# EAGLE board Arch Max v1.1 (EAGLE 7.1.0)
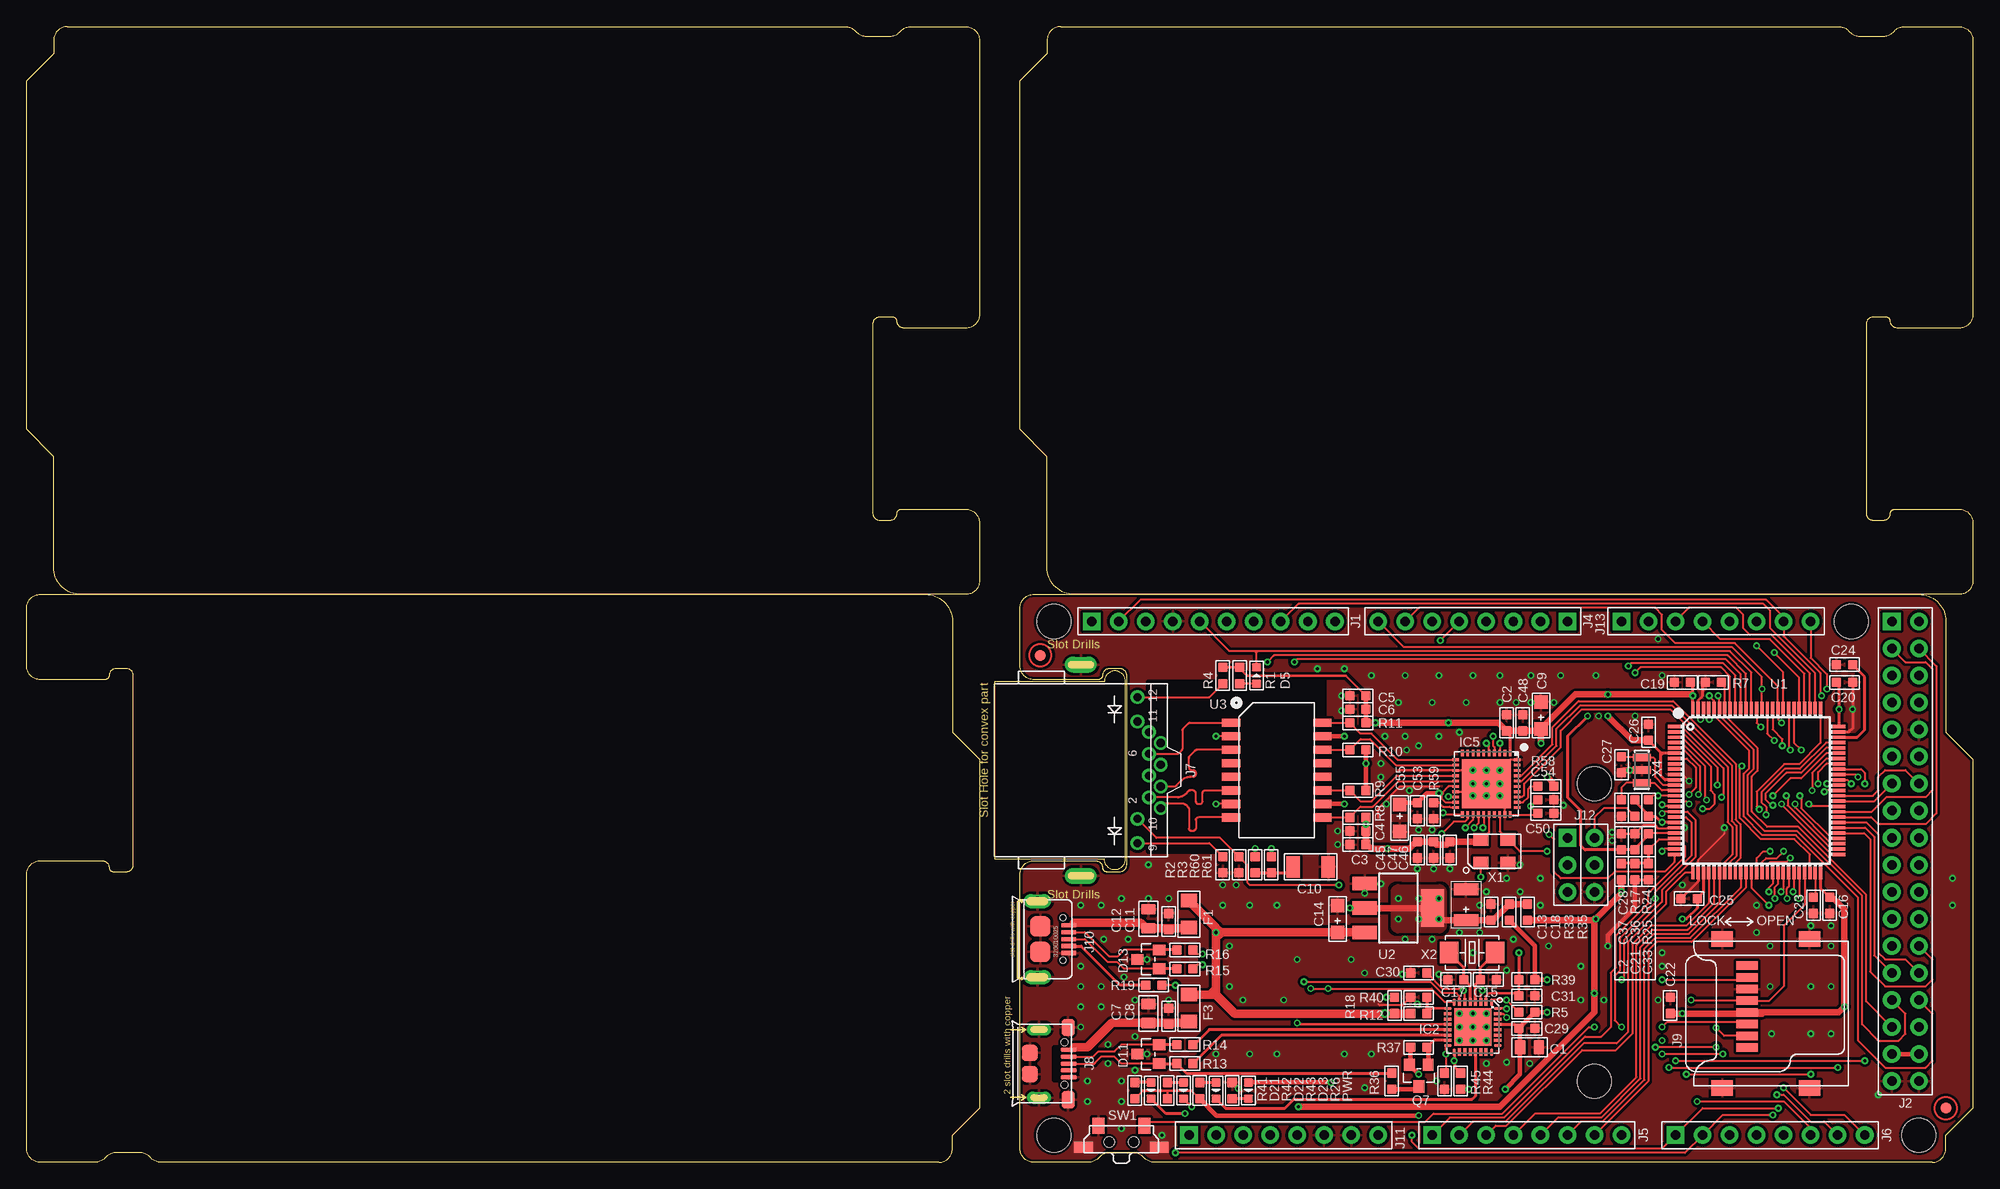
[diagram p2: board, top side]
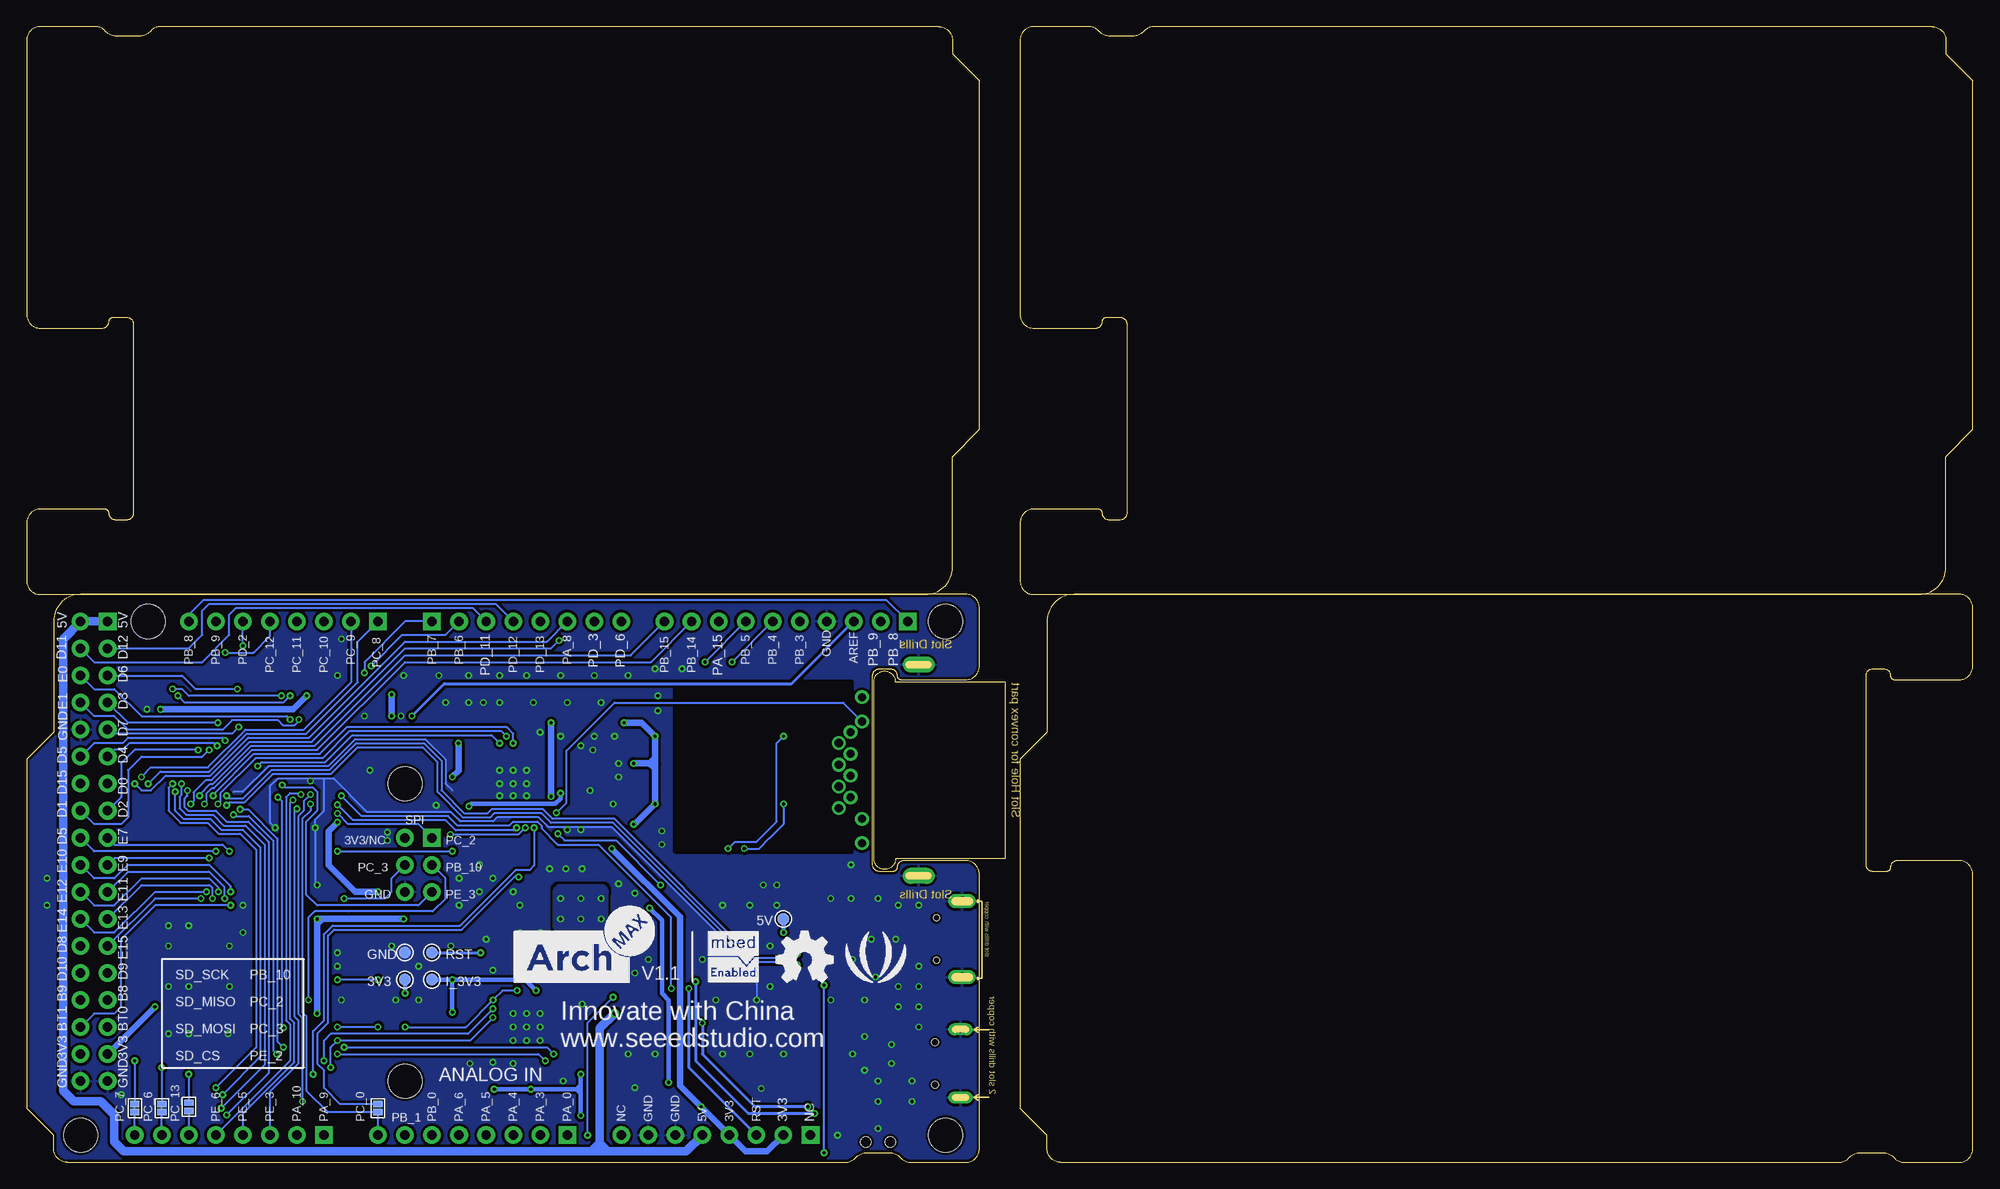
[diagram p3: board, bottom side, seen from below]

Size 182.88 x 106.68 mm. Coordinates in mm from the lower left corner, seen from the top.
Outline: 136 segments
Copper layers (1*16): Top 0.035mm / dielectric 1.5mm / Bottom 0.035mm
Design rules "SeeedStudio_2layer_DRU_no_angle_20140221 *": minimum track width 6mil, minimum drill 12mil, track to track 6mil, track to pad 6mil, pad to pad 6mil, via to via 6mil, smd to smd 0mil, copper to edge 10mil, drill to drill 10mil, minimum pad ring 10mil, minimum via ring 6mil, stop-mask expansion 2mil, vias tented up to drill 100mil, thermal gap 10mil
Net classes: 0 default: width 0.102 mm, drill 0.203 mm, clearance 0.102 mm
Holes 3.2 mm at 171.45,50.8 177.8,2.54 147.32,35.56 96.52,50.8 96.52,2.54 147.32,7.62
Holes 1.91 mm at 2.54,-6.35 180.34,-6.35 2.54,113.03 180.34,113.03
tRestrict: area 105.4,29.2 to 121.9,45.1
bRestrict: area 105.4,29.2 to 121.9,45.1

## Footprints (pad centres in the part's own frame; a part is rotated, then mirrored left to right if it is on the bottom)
TP_4545 = smd 1.143 x 1.143: T 0,0
C0805 = smd 1.016 x 1.397: 1 -0.889,0; 2 0.889,0
C0603 = smd 0.889 x 0.889: 1 -0.762,0; 2 0.762,0
AVX-A = smd 1.27 x 1.27: + -1.27,0; - 1.27,0
C1206 = smd 1.27 x 2.032: 1 -1.651,0; 2 1.651,0
AVX-B = smd 1.143 x 2.286: + -1.46,0; - 1.46,0
LED-0603 = smd 0.762 x 0.889: + -0.762,0; - 0.762,0
SOT23 = smd 1.016 x 1.143: 1 -0.889,-1.016; 2 0.889,-1.016; 3 0,1.016
F1206 = smd 1.27 x 1.524: 1 -1.27,0; 2 1.27,0
MBED-ICS_HVQFN33 = smd 0.7 x 0.28: 1 -2.35,1.75; 2 -2.35,1.25; 3 -2.35,0.75; 4 -2.35,0.25; 5 -2.35,-0.25; 6 -2.35,-0.75; 7 -2.35,-1.25; 8 -2.35,-1.75; 17 2.35,-1.75; 18 2.35,-1.25; 19 2.35,-0.75; 20 2.35,-0.25; 21 2.35,0.25; 22 2.35,0.75; 23 2.35,1.25; 24 2.35,1.75 | smd 0.28 x 0.7: 9 -1.75,-2.35; 10 -1.25,-2.35; 11 -0.75,-2.35; 12 -0.25,-2.35; 13 0.25,-2.35; 14 0.75,-2.35; 15 1.25,-2.35; 16 1.75,-2.35; 25 1.75,2.35; 26 1.25,2.35; 27 0.75,2.35; 28 0.25,2.35; 29 -0.25,2.35; 30 -0.75,2.35; 31 -1.25,2.35; 32 -1.75,2.35 | smd 3.5 x 3.5: EXP 0,0
LLP-40 = smd 0.25 x 0.6: 1 2.25,2.9; 2 1.75,2.9; 3 1.25,2.9; 4 0.75,2.9; 5 0.25,2.9; 6 -0.25,2.9; 7 -0.75,2.9; 8 -1.25,2.9; 9 -1.75,2.9; 10 -2.25,2.9; 21 -2.25,-2.9; 22 -1.75,-2.9; 23 -1.25,-2.9; 24 -0.75,-2.9; 25 -0.25,-2.9; 26 0.25,-2.9; 27 0.75,-2.9; 28 1.25,-2.9; 29 1.75,-2.9; 30 2.25,-2.9 | smd 0.6 x 0.25: 11 -2.9,2.25; 12 -2.9,1.75; 13 -2.9,1.25; 14 -2.9,0.75; 15 -2.9,0.25; 16 -2.9,-0.25; 17 -2.9,-0.75; 18 -2.9,-1.25; 19 -2.9,-1.75; 20 -2.9,-2.25; 31 2.9,-2.25; 32 2.9,-1.75; 33 2.9,-1.25; 34 2.9,-0.75; 35 2.9,-0.25; 36 2.9,0.25; 37 2.9,0.75; 38 2.9,1.25; 39 2.9,1.75; 40 2.9,2.25 | smd 4.6 x 4.6: DAP 0,0
10P-2.54-65/35MIL = drill 0.889 pad 1.651 square: 1 0,11.43 | drill 0.889 pad 1.651: 2 0,8.89; 3 0,6.35; 4 0,3.81; 5 0,1.27; 6 0,-1.27; 7 0,-3.81; 8 0,-6.35; 9 0,-8.89; 10 0,-11.43
2.54-2X18P = drill 0.889 pad 1.651 square: 1 -1.27,21.59 | drill 0.889 pad 1.651: 2 -1.27,19.05; 3 -1.27,16.51; 4 -1.27,13.97; 5 -1.27,11.43; 6 -1.27,8.89; 7 -1.27,6.35; 8 -1.27,3.81; 9 -1.27,1.27; 10 -1.27,-1.27; 11 -1.27,-3.81; 12 -1.27,-6.35; 13 -1.27,-8.89; 14 -1.27,-11.43; 15 -1.27,-13.97; 16 -1.27,-16.51; 17 -1.27,-19.05; 18 -1.27,-21.59; 19 1.27,-21.59; 20 1.27,-19.05; 21 1.27,-16.51; 22 1.27,-13.97; 23 1.27,-11.43; 24 1.27,-8.89; 25 1.27,-6.35; 26 1.27,-3.81; 27 1.27,-1.27; 28 1.27,1.27; 29 1.27,3.81; 30 1.27,6.35; 31 1.27,8.89; 32 1.27,11.43; 33 1.27,13.97; 34 1.27,16.51; 35 1.27,19.05; 36 1.27,21.59
CK_1X8 = drill 0.889 pad 1.651 square: 1 0,8.89 | drill 0.889 pad 1.651: 2 0,6.35; 3 0,3.81; 4 0,1.27; 5 0,-1.27; 6 0,-3.81; 7 0,-6.35; 8 0,-8.89
RJ45-MJ88-BX11-RVSL2 = drill 0.762 pad 1.27: 1 3.57,7.5; 2 2.55,6.4; 3 1.53,7.5; 4 0.51,6.4; 5 -0.51,7.5; 6 -1.53,6.4; 7 -2.55,7.5; 8 -3.57,6.4; 9 6.86,5.32; 10 4.57,5.32; 11 -4.57,5.32; 12 -6.86,5.32 | drill 0.6 pad 1.5 long: 13 -9.92,0; 14 9.92,0
MICRO-USB = smd 0.381 x 1.524: 1 -1.3,-0.25; 2 -0.65,-0.25; 3 0,-0.25; 4 0.65,-0.25; 5 1.3,-0.25 | smd 1.6 x 1.2: S1 -3.4,-0.3; S6 3.4,-0.3 | drill 0.635 pad 1.143 long: S2 -3.2,-3.048; S5 3.2,-3.048 | smd 1.5 x 1.5: S3 -1,-3.9; S4 1,-3.9 | hole 0.635: -2,-0.65; 2,-0.65
8P-SMD = smd 0.8 x 2.008: 1 -3.198,0.254; 2 -2.098,0.254; 3 -0.998,0.254; 4 0.102,0.254; 5 1.202,0.254; 6 2.302,0.254; 7 3.402,0.254; 8 4.502,0.254 | smd 1.45 x 2: 9 -7.002,2.6; 10 7.002,2.6; 11 -7.002,-5.598; 12 7.002,-5.598
MICRO-USB-5P-AB = smd 0.4 x 1.35: 1 -1.3,2.675; 2 -0.65,2.675; 3 0,2.675; 4 0.65,2.675; 5 1.3,2.675 | smd 1.9 x 1.9: P1 -1.2,0; P2 1.2,0 | drill 0.8 pad 1.2 long: P3 -3.575,-0.265; P4 3.575,-0.265 | hole 0.55: -2,2.15; 2,2.15
2X3P-2.54-65/35MIL = drill 0.889 pad 1.651 square: 1 -1.27,2.54 | drill 0.889 pad 1.651: 2 -1.27,0; 3 -1.27,-2.54; 4 1.27,-2.54; 5 1.27,0; 6 1.27,2.54
L0603 = smd 0.889 x 0.889: 1 -0.762,0; 2 0.762,0
2P-SMD-1.78X1.27 = smd 0.889 x 0.61: 1 0,0.381; 2 0,-0.381
ROUND-MARK-1.0 = smd 1.016 x 1.016: P$1 0,0
R0603 = smd 0.889 x 0.889: 1 -0.762,0; 2 0.762,0
4P-SMD-7X3.5X3.5H = smd 1.143 x 1.524: 1 -2.159,1.524; 2 2.159,1.524 | smd 1.778 x 1.016: S1 -3.556,-0.508; S2 3.556,-0.508 | hole 0.95: -1.15,0; 1.15,0
LQFP100 = smd 1.2 x 0.32: 1 -7.75,6; 2 -7.75,5.5; 3 -7.75,5; 4 -7.75,4.5; 5 -7.75,4; 6 -7.75,3.5; 7 -7.75,3; 8 -7.75,2.5; 9 -7.75,2; 10 -7.75,1.5; 11 -7.75,1; 12 -7.75,0.5; 13 -7.75,0; 14 -7.75,-0.5; 15 -7.75,-1; 16 -7.75,-1.5; 17 -7.75,-2; 18 -7.75,-2.5; 19 -7.75,-3; 20 -7.75,-3.5; 21 -7.75,-4; 22 -7.75,-4.5; 23 -7.75,-5; 24 -7.75,-5.5; 25 -7.75,-6; 51 7.75,-6; 52 7.75,-5.5; 53 7.75,-5; 54 7.75,-4.5; 55 7.75,-4; 56 7.75,-3.5; 57 7.75,-3; 58 7.75,-2.5; 59 7.75,-2; 60 7.75,-1.5; 61 7.75,-1; 62 7.75,-0.5; 63 7.75,0; 64 7.75,0.5; 65 7.75,1; 66 7.75,1.5; 67 7.75,2; 68 7.75,2.5; 69 7.75,3; 70 7.75,3.5; 71 7.75,4; 72 7.75,4.5; 73 7.75,5; 74 7.75,5.5; 75 7.75,6 | smd 0.32 x 1.2: 26 -6,-7.75; 27 -5.5,-7.75; 28 -5,-7.75; 29 -4.5,-7.75; 30 -4,-7.75; 31 -3.5,-7.75; 32 -3,-7.75; 33 -2.5,-7.75; 34 -2,-7.75; 35 -1.5,-7.75; 36 -1,-7.75; 37 -0.5,-7.75; 38 0,-7.75; 39 0.5,-7.75; 40 1,-7.75; 41 1.5,-7.75; 42 2,-7.75; 43 2.5,-7.75; 44 3,-7.75; 45 3.5,-7.75; 46 4,-7.75; 47 4.5,-7.75; 48 5,-7.75; 49 5.5,-7.75; 50 6,-7.75; 76 6,7.75; 77 5.5,7.75; 78 5,7.75; 79 4.5,7.75; 80 4,7.75; 81 3.5,7.75; 82 3,7.75; 83 2.5,7.75; 84 2,7.75; 85 1.5,7.75; 86 1,7.75; 87 0.5,7.75; 88 0,7.75; 89 -0.5,7.75; 90 -1,7.75; 91 -1.5,7.75; 92 -2,7.75; 93 -2.5,7.75; 94 -3,7.75; 95 -3.5,7.75; 96 -4,7.75; 97 -4.5,7.75; 98 -5,7.75; 99 -5.5,7.75; 100 -6,7.75
SOT-223 = smd 1.27 x 2.286: 1 -2.286,-3.175; 2 0,-3.175; 3 2.286,-3.175 | smd 3.556 x 2.159: TER 0,3.175
SOIC16-9.53 = smd 0.762 x 1.714: 1 -4.445,-4.286; 2 -3.175,-4.286; 3 -1.905,-4.286; 4 -0.635,-4.286; 5 0.635,-4.286; 6 1.905,-4.286; 7 3.175,-4.286; 8 4.445,-4.286; 9 4.445,4.286; 10 3.175,4.286; 11 1.905,4.286; 12 0.635,4.286; 13 -0.635,4.286; 14 -1.905,4.286; 15 -3.175,4.286; 16 -4.445,4.286
4P-SMD-5X3.2 = smd 1.4 x 1.2: 1 -1.27,-1.1; 2 1.27,-1.1; 3 1.27,1.1; 4 -1.27,1.1
2P-SMD-5X3.2 = smd 1.778 x 2.032: 1 -2.159,0; 2 2.159,0
3P-SMD-3.6X1.3 = smd 0.7 x 1.7: 1 -1.2,0; 2 0,0; 3 1.2,0

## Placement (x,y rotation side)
3V3  NC  [TP_4545]  147.32,17.14 270 bottom
5V  NC  [TP_4545]  111.76,22.86 270 bottom
C1  10uF  [C0805]  141.22,10.79 180 top
C2  100nF  [C0603]  139.06,41.27 270 top
C3  100nF  [C0603]  125.09,29.84 180 top
C4  100nF  [C0603]  125.09,31.11 180 top
C5  100nF  [C0603]  125.09,43.81 180 top
C6  100nF  [C0603]  125.09,42.55 180 top
C7  10uF  [C0805]  105.41,13.97 90 top
C8  100nF  [C0603]  107.31,13.72 90 top
C9  16V 10uF  [AVX-A]  142.3,41.97 90 top
C10  1000v_1nF  [C1206]  120.65,27.75 180 top
C11  100nF  [C0603]  107.31,22.61 90 top
C12  10uF  [C0805]  105.41,22.86 90 top
C13  10V 47uF  [AVX-B]  135.25,24.19 90 top
C14  10uF/16v  [AVX-A]  123.19,22.86 90 top
C15  18pF  [C0603]  137.35,17.14 180 top
C16  100nF  [C0603]  169.42,24.13 90 top
C17  18pF  [C0603]  134.3,17.14 0 top
C18  100nF  [C0603]  137.6,23.5 270 top
C19  100nF  [C0603]  155.57,45.09 0 top
C20  100nF  [C0603]  170.81,45.09 180 top
C21  100nF  [C0603]  151.13,27.3 90 top
C22  100nF  [C0603]  154.43,14.73 90 top
C23  2.2uF  [C0603]  167.89,24.13 90 top
C24  2.2uF  [C0603]  170.81,46.74 0 top
C25  100nF  [C0603]  156.21,24.77 0 top
C26  100nF  [C0603]  152.4,40.39 270 top
C27  DNP  [C0603]  149.86,37.34 90 top
C28  DNP  [C0603]  149.86,33.27 90 top
C29  100nF  [C0603]  140.97,12.57 180 top
C30  100nF  [C0603]  130.81,17.78 0 top
C31  100nF  [C0603]  140.97,15.62 180 top
C33  1uF  [C0603]  152.4,27.3 90 top
C36  1uF  [C0603]  151.13,30.1 270 top
C37  100nF  [C0603]  149.86,30.1 270 top
C45  100nF  [C0603]  130.68,29.34 90 top
C46  100nF  [C0603]  133.73,29.34 90 top
C47  100nF  [C0603]  132.21,29.34 270 top
C48  100nF  [C0603]  140.59,41.27 90 top
C50  100nF  [C0603]  142.75,32.77 0 top
C53  100nF  [C0603]  130.68,33.02 90 top
C54  100nF  [C0603]  142.75,34.04 180 top
C55  16V 10uF  [AVX-A]  129.03,32.32 270 top
D5  GREEN  [LED-0603]  115.57,45.72 90 top
D11  CESD3V3AP  [SOT23]  105.41,10.16 90 top
D13  CESD3V3AP  [SOT23]  105.41,19.05 90 top
D21  RED  [LED-0603]  105.66,6.73 270 top
D22  BULE  [LED-0603]  108.71,6.73 270 top
D23  YELLOW  [LED-0603]  111.76,6.73 270 top
F1  PPTC_750mA  [F1206]  109.22,23.3 90 top
F3  PPTC_750mA  [F1206]  109.22,14.48 90 top
GND  NC  [TP_4545]  147.32,19.68 270 bottom
I_3V3  NC  [TP_4545]  144.78,17.14 270 bottom
IC2  LPC11U35FHI33/501  [MBED-ICS_HVQFN33]  135.89,12.7 270 top
IC5  DP83848J  [LLP-40]  137.16,35.56 0 top
J1  320030059  [10P-2.54-65/35MIL]  111.51,50.8 90 top
J2  DNP/2.54 Female 2*18p  [2.54-2X18P]  176.53,29.21 0 top
J4  2.54 female 8p  [CK_1X8]  135.89,50.8 270 top
J5  2.54 female 8p  [CK_1X8]  140.97,2.54 90 top
J6  2.54 female 8p  [CK_1X8]  163.83,2.54 90 top
J7  RJ45-MJ88-BX11-RVSL2  [RJ45-MJ88-BX11-RVSL2]  99.06,36.83 270 top
J8  340005001  [MICRO-USB]  98.17,9.27 270 top
J9  320090002  [8P-SMD]  161.93,13.97 90 top
J10  320010025  [MICRO-USB-5P-AB]  95.25,20.95 270 top
J11  2.54 female 8p  [CK_1X8]  118.11,2.54 90 top
J12  320020027  [2X3P-2.54-65/35MIL]  146.05,27.94 0 top
J13  2.54 female 8p  [CK_1X8]  158.75,50.8 90 top
L2  120R-500mA  [L0603]  149.86,27.3 270 top
P1  NC  [2P-SMD-1.78X1.27]  167.64,5.21 180 bottom
P2  NC  [ROUND-MARK-1.0]  not placed on the board
P3  NC  [ROUND-MARK-1.0]  not placed on the board
P4  NC  [ROUND-MARK-1.0]  not placed on the board
P5  NC  [2P-SMD-1.78X1.27]  149.86,5.08 180 bottom
P6  NC  [ROUND-MARK-1.0]  180.34,5.08 0 top
P7  NC  [ROUND-MARK-1.0]  95.25,47.62 0 top
P8  NC  [ROUND-MARK-1.0]  not placed on the board
P9  NC  [2P-SMD-1.78X1.27]  170.18,5.08 0 bottom
P10  NC  [2P-SMD-1.78X1.27]  172.72,5.08 180 bottom
PWR  Green  [LED-0603]  114.81,6.73 270 top
Q7  CJ2305  [SOT23]  130.81,8.13 180 top
R1  470R  [R0603]  113.98,45.72 90 top
R2  470R  [R0603]  112.39,27.94 90 top
R3  2.2K  [R0603]  113.92,27.94 90 top
R4  470R  [R0603]  112.39,45.72 270 top
R5  DNP  [R0603]  140.97,14.1 0 top
R7  10K  [R0603]  158.5,45.09 0 top
R8  49.9R_1%  [R0603]  125.09,32.38 180 top
R9  49.9R_1%  [R0603]  125.09,34.92 0 top
R10  49.9R_1%  [R0603]  125.09,38.73 180 top
R11  49.9R_1%  [R0603]  125.09,41.27 0 top
R12  10k  [R0603]  130.81,13.97 180 top
R13  33R  [R0603]  108.84,9.27 180 top
R14  33R  [R0603]  108.84,11.05 180 top
R15  33R  [R0603]  108.84,18.16 180 top
R16  33R  [R0603]  108.84,19.94 180 top
R17  DNP  [R0603]  151.13,33.27 90 top
R18  10k  [R0603]  128.52,14.73 270 top
R19  0R  [R0603]  105.92,16.64 180 top
R24  10K  [R0603]  152.4,33.27 270 top
R25  0R  [R0603]  152.4,30.1 270 top
R26  470R  [R0603]  113.28,6.73 270 top
R33  0R  [R0603]  139.32,23.5 270 top
R35  0R  [R0603]  141.03,23.5 90 top
R36  1.5k  [R0603]  128.27,7.62 90 top
R37  DNP  [R0603]  130.81,10.79 180 top
R39  10k  [R0603]  140.97,17.14 0 top
R40  100k  [R0603]  130.81,15.49 0 top
R41  470R  [R0603]  104.14,6.73 270 top
R42  470R  [R0603]  107.19,6.73 270 top
R43  470R  [R0603]  110.24,6.73 270 top
R44  DNP  [R0603]  134.75,7.62 270 top
R45  DNP  [R0603]  133.22,7.62 90 top
R58  2.2K  [R0603]  142.75,35.31 180 top
R59  4.87K_1%  [R0603]  132.21,33.02 270 top
R60  75R  [R0603]  115.44,27.94 90 top
R61  75R  [R0603]  116.97,27.94 90 top
RST  NC  [TP_4545]  144.78,19.68 0 bottom
SW1  BUTTON-4P-REINFORCE'TS-1188E'  [4P-SMD-7X3.5X3.5H]  102.87,1.91 0 top
U1  STM32F407VET6  [LQFP100]  162.56,34.92 0 top
U2  CJT1117-3.3  [SOT-223]  128.91,23.88 270 top
U3  HX1198NL  [SOIC16-9.53]  117.47,36.83 270 top
U$1  [SEEEDSTUDIO-PCB-FRAME]  not placed on the board
U$2  [SEEEDSTUDIO-PCB-FRAME]  not placed on the board
U$3  [SEEEDSTUDIO-PCB-FRAME]  not placed on the board
U$4  [SEEEDSTUDIO-PCB-FRAME]  not placed on the board
U$5  [SEEEDSTUDIO-PCB-FRAME]  not placed on the board
X1  50MHz/052012001  [4P-SMD-5X3.2]  137.92,29.21 0 top
X2  12MHz/050016001  [2P-SMD-5X3.2]  135.83,19.68 0 top
X4  8MHz  [3P-SMD-3.6X1.3]  151.76,36.83 270 top

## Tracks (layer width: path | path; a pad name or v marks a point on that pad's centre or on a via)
50MHZ  (via drill 0.3 pad 0.64)
  Top 0.203: IC5.28 138.41,31.09 X1.3 140.29,29.21 v142.88,29.21 | U1.24 153.88,29.43 v153.67,29.21
  Bottom 0.203: v153.67,29.21 v142.88,29.21
+3.3V  (via drill 0.3 pad 0.64)
  Top 0.203: IC5.18 133.65,34.31 v133.6,34.35 | IC5.26 137.41,32.7 137.41,30.99 136.74,30.31 X1.4 | 170.31,45.08 C20.2 | 151.13,33.91 R17.2
  Top 0.254: R4.1 R1.2 113.98,46.42 114.68,45.72 123.95,45.72 C5.1
  Top 0.305: U1.28 157.56,25.35 C25.2 156.97,23.88 155.96,22.86 v155.57,22.86 | U1.100 v156.56,43.81 156.56,44.86 C19.2 | U1.75 v170.31,42.54 170.31,45.08 | R24.2 152.4,32.38 | R17.2 151.13,34.16 | U1.50 168.56,25.75 C16.2 | IC5.1 139.41,40.26 | 139.41,40.26 139.41,40.8 | 151.13,33.91 152.4,32.64 R24.2 | C2.2 139.16,40.51 139.41,40.26 | U1.6 153.74,38.42 | 153.74,38.42 153.6,38.42 | 153.6,38.42 153.54,38.48 | 153.54,38.48 C26.2 | U1.11 153.94,35.92 153.54,36.32 153.54,38.23 | 153.54,38.23 153.54,38.37 | 153.54,38.37 153.6,38.42 | 153.54,38.37 153.54,38.48 | U1.19 153.66,31.93 | R24.2 153.03,32.51 153.62,31.93 153.66,31.93 | 153.74,38.42 153.54,38.23 | 153.66,31.93 v153.67,31.94
  Top 0.406: C5.1 C6.1 R11.2 | R10.1 v125.86,37.47 R9.2 | U3.10 v123.82,33.66 | v123.82,40.01 U3.15 | 130.43,29.84 C45.2 130.56,30.1 | J2.20 J2.17 | C25.2 156.97,24.64 | 136.55,30.2 X1.4
  Top 0.61: R11.2 v126.75,41.27 v133.6,41.27 138.3,41.27 C2.2 C48.1 142.11,40.51 C9.+ | C16.2 169.67,24.89 170.81,23.75 v170.81,14.61 170.28,14.07 163.19,14.07 | J9.4 163.19,14.07 | 163.19,14.07 163.09,13.97 v155.57,13.97 C22.1 | C9.+ v142.3,39.37 | C9.+ 145.54,43.94 v148.59,43.94 156.43,43.94 v156.56,43.81 | v147.45,22.86 147.32,22.86 147.32,22.73 | 147.32,22.48 v147.32,15.88 147.32,14.1 138.43,5.21 v119.51,5.21 | 147.32,22.48 147.32,22.73 | 147.32,22.48 147.07,22.73 | R8.1 v125.86,31.75 C4.1 125.86,29.97 | 125.86,29.97 C3.1 | 125.86,29.97 126.36,29.46 v127.89,29.46 129.92,29.46 130.56,30.1 | C45.2 C47.1 132.46,29.84 133.48,29.84 C46.2 136.44,30.1 136.55,30.2 | L2.2 v149.86,25.4 149.86,25.27 v147.45,22.86 | R35.1 147.32,22.73 | 147.32,22.73 v147.45,22.86 | R58.1 143.51,35.56 v142.88,36.2 | C26.2 150.88,39.62 v148.59,41.91
  Bottom 0.406: 3V3.T v147.32,15.88
  Bottom 0.61: 123.82,37.47 v123.82,33.66 125.73,31.75 v125.86,31.75 | 123.82,37.47 v123.82,40.01 125.09,41.27 v126.75,41.27 | v125.86,37.47 124.46,37.47 | 124.46,37.47 123.82,37.47 | J2.17 v170.81,14.61 | 124.46,37.47 arc-45 124.24,37.55 123.95,37.85 | 124.46,37.47 arc45 124.24,37.38 123.95,37.08 | v170.31,42.54 157.83,42.54 v156.56,43.81 | v127.89,29.46 121.48,23.05 121.48,7.18 v119.51,5.21 J11.4 115.32,1.02 113.28,1.02 J11.2 | v133.6,34.35 v133.6,41.27 | v142.3,39.37 142.3,36.77 v142.88,36.2 | v148.59,41.91 v148.59,43.94 | v153.67,31.94 154.5,31.11 154.5,27.88 152.02,25.4 v149.86,25.4 | v147.45,22.86 155.07,22.86 | 155.07,22.86 155.45,22.86 | v155.57,13.97 155.57,22.35 | 155.57,22.35 v155.57,22.86 | 155.07,22.86 155.57,22.35
AREF  (via drill 0.3 pad 0.64)
  Top 0.203: U1.21 152.72,30.93 152.65,30.86 R25.1
  Top 0.305: R25.1 152.4,30.73 151.13,29.46 C36.2 C37.2 146.43,29.34 146.05,29.72 146.05,33.02 144.78,34.29 144.78,40.01 v146.69,41.91
  Bottom 0.305: v146.69,41.91 143.64,44.96 111,44.96 J1.3
BOOT0
  Top 0.203: J2.16 172.85,15.11 172.85,25.15 166.5,31.5 163.54,31.5 162.11,32.93 162.11,36.25 162.62,36.77 162.62,38.92 159.56,41.99 U1.94 159.56,45.04 159.51,45.09 R7.2
BOOT1  (via drill 0.3 pad 0.64)
  Top 0.203: U1.37 162.06,25.77 v163.7,24.13
  Bottom 0.203: v163.7,24.13 170.81,24.13 173.99,20.95 173.99,14.61 174.62,13.97 176.53,13.97 J2.21
DB_RX  (via drill 0.3 pad 0.64)
  Top 0.203: v154.94,9.53 v172.72,9.53
  Top 0.254: IC2.32 139.03,14.45 v139.06,14.41
  Bottom 0.203: v139.06,14.41 141.41,12.06 154.31,12.06 154.94,11.43 v154.94,9.53 | v172.72,9.53 P10.2
DB_TX  (via drill 0.3 pad 0.64)
  Top 0.203: IC2.31 138.7,13.95 v139.06,13.59 | v154.31,8.89 v170.18,8.89
  Bottom 0.203: v139.06,13.59 141.22,11.43 v153.67,11.43 154.31,10.79 v154.31,8.89 | v170.18,8.89 P9.1
ETH_CRS_DV
  Top 0.203: U1.32 159.56,28.18 160.27,28.89 160.27,31.5 159.83,31.94 159.83,37.15 154.43,42.55 146.15,42.55 144.14,40.54 144.14,38.99 140.72,35.56 140.72,34.54 140.48,34.31 IC5.33
ETH_MDC  (via drill 0.3 pad 0.64)
  Top 0.203: U1.16 153.84,33.42 v153.67,33.59 | IC5.25 136.91,31.5 v136.84,31.43
  Bottom 0.203: v136.84,31.43 137.1,31.18 142.56,31.18 143.51,32.13 152.21,32.13 v153.67,33.59
ETH_MDIO  (via drill 0.3 pad 0.64)
  Top 0.203: IC5.24 136.41,31.83 v136.02,31.43 | U1.25 154.81,28.19 153.92,27.3 149.22,27.3 148.59,26.67 144.14,26.67 143.51,27.3 143.51,30.35 v143.06,30.8
  Bottom 0.203: v136.02,31.43 136.65,30.8 v143.06,30.8
ETH_RX_D0
  Top 0.203: IC5.36 140.46,35.81 143.76,39.12 143.76,40.7 145.99,42.93 154.58,42.93 160.21,37.3 160.21,32.07 160.66,31.62 160.66,28.77 160.06,28.17 U1.33
ETH_RX_D1
  Top 0.203: U1.34 160.56,28.1 161.04,28.57 161.04,31.75 160.59,32.19 160.59,37.43 154.71,43.31 145.81,43.31 143.38,40.88 143.38,39.24 140.45,36.31 IC5.37
ETH_TX_D0  (via drill 0.3 pad 0.64)
  Top 0.203: U1.51 169.58,28.93 164.91,33.59 v164.91,33.66 | v137.79,40.01 137.79,39.12 137.92,38.99 137.92,38.47 IC5.4
  Bottom 0.203: v164.91,33.66 164.68,33.88 164.68,34.65 161.36,37.97 155.07,37.97 152.53,40.51 138.3,40.51 v137.79,40.01
ETH_TX_D1  (via drill 0.3 pad 0.64)
  Top 0.203: U1.52 169.58,29.43 165.48,33.53 165.48,34.29 v165.35,34.42 | IC5.5 137.41,39.12 v137.16,39.37
  Bottom 0.203: v137.16,39.37 137.16,40.26 137.79,40.89 152.78,40.89 155.32,38.35 161.54,38.35 165.35,34.54 v165.35,34.42
ETH_TX_EN  (via drill 0.3 pad 0.64)
  Top 0.203: U1.48 167.56,28.91 166.12,30.35 162.96,30.35 160.97,32.35 160.97,37.02 v161.16,37.21 | v138.43,39.37 138.43,38.48 IC5.3
  Bottom 0.203: v161.16,37.21 160.78,37.59 154.81,37.59 152.27,40.13 139.19,40.13 v138.43,39.37
FSMC_D0
  Top 0.203: U1.61 173.62,33.92 J2.7
FSMC_D1
  Top 0.203: U1.62 173.49,34.42 173.99,34.92 173.99,36.2 174.62,36.83 176.53,36.83 J2.30
FSMC_D2  (via drill 0.3 pad 0.64)
  Top 0.203: U1.81 166.06,39.43 v166.75,38.73
  Bottom 0.203: J2.8 173.99,34.29 173.99,37.47 172.72,38.73 v166.75,38.73
FSMC_D3  (via drill 0.3 pad 0.64)
  Top 0.203: U1.82 165.56,38.91 v165.74,38.73
  Bottom 0.203: J2.29 176.53,31.75 173.99,31.75 173.35,32.38 173.35,36.83 172.08,38.1 166.37,38.1 v165.74,38.73
FSMC_D4  (via drill 0.3 pad 0.64)
  Top 0.203: U1.38 162.56,28.57 163.19,29.21 v163.83,29.21
  Bottom 0.203: J2.9 174.62,29.84 164.46,29.84 v163.83,29.21
FSMC_D5  (via drill 0.3 pad 0.64)
  Top 0.203: U1.39 163.06,28.19 163.45,28.57 164.46,28.57 v165.1,29.21
  Bottom 0.203: v165.1,29.21 176.53,29.21 J2.28
FSMC_D6  (via drill 0.3 pad 0.64)
  Top 0.203: U1.40 163.56,27.92 163.83,28.19 165.35,28.19 v165.74,28.57
  Bottom 0.203: v165.74,28.57 174.62,28.57 J2.10
FSMC_D7  (via drill 0.3 pad 0.64)
  Top 0.203: v163.7,25.4 163.7,25.78 164.06,26.14 U1.41
  Bottom 0.203: J2.27 176.53,26.67 174.62,26.67 173.35,27.94 165.74,27.94 163.7,25.91 v163.7,25.4
FSMC_D8  (via drill 0.3 pad 0.64)
  Top 0.203: v164.27,24.77 164.27,25.84 164.56,26.13 U1.42
  Bottom 0.203: v164.27,24.77 164.27,25.84 165.74,27.3 173.35,27.3 J2.11
FSMC_D9  (via drill 0.3 pad 0.64)
  Top 0.203: U1.43 165.06,25.61 v164.85,25.4
  Bottom 0.203: J2.26 176.53,24.13 174.62,24.13 172.08,26.67 165.74,26.67 164.85,25.78 v164.85,25.4
FSMC_D10  (via drill 0.3 pad 0.64)
  Top 0.203: v165.42,24.77 165.42,25.72 165.56,25.86 U1.44
  Bottom 0.203: v165.42,24.77 165.42,25.72 165.74,26.04 172.08,26.04 J2.12
FSMC_D11  (via drill 0.3 pad 0.64)
  Top 0.203: U1.45 166.06,25.47 v165.99,25.4
  Bottom 0.203: J2.25 176.53,21.59 174.62,21.59 170.81,25.4 v165.99,25.4
FSMC_D12  (via drill 0.3 pad 0.64)
  Top 0.203: v166.5,24.77 166.62,24.89 166.62,27.11 U1.46
  Bottom 0.203: v166.5,24.77 170.81,24.77 J2.13
FSMC_D13
  Top 0.203: U1.55 172.66,30.93 173.23,30.35 173.23,17.91 174.62,16.51 178.44,16.51 179.07,17.14 179.07,19.05 J2.24
FSMC_D14
  Top 0.203: U1.56 172.75,31.43 173.61,30.57 173.61,19.43 J2.14
FSMC_D15
  Top 0.203: U1.57 172.86,31.93 173.99,30.79 173.99,19.68 174.62,19.05 176.53,19.05 J2.23
FSMC_NBL0  (via drill 0.3 pad 0.64)
  Top 0.203: U1.97 158.06,41.65 v158.12,41.59
  Bottom 0.203: J2.34 176.53,44.45 174.62,44.45 172.08,41.91 158.43,41.91 v158.12,41.59
FSMC_NBL1  (via drill 0.3 pad 0.64)
  Top 0.203: U1.98 157.56,41.86 v157.29,41.59
  Bottom 0.203: J2.33 176.53,41.91 174.62,41.91 173.35,40.64 164.46,40.64 163.58,41.53 159.26,41.53 158.75,41.02 157.73,41.02 157.29,41.47 v157.29,41.59
FSMC_NE1/NCE2  (via drill 0.3 pad 0.64)
  Top 0.203: U1.88 | U1.88 162.56,42.74 162.5,42.8 | U1.88 162.56,41.27 v162.94,40.89
  Bottom 0.203: J2.5 174.88,40.26 163.58,40.26 v162.94,40.89
FSMC_NOE  (via drill 0.3 pad 0.64)
  Top 0.203: U1.85 164.06,40.66 164.97,39.75 v164.97,39.12
  Bottom 0.203: J2.6 174.62,38.73 173.86,38.73 173.23,39.37 165.23,39.37 v164.97,39.12
FSMC_NWE  (via drill 0.3 pad 0.64)
  Top 0.203: 163.58,42.67 163.57,42.67 U1.86 163.56,40.27 v164.21,39.62
  Bottom 0.203: J2.31 176.53,39.37 173.86,39.37 173.35,39.88 164.46,39.88 v164.21,39.62
GND  (via drill 0.3 pad 0.64)
  Top 0.203: 128.91,36.83 128.93,36.81 IC5.13 135.87,36.81 135.87,37.45 | 132.72,35.31 129.03,35.31 127,33.27 127,32.38 | C37.1 C36.1 151.95,31.69 152.97,31.69 153.29,31.37 154.75,31.37 U1.20 155.76,31.43 v155.76,31.43 | IC5.17 135.37,34.81 | IC5.29 138.91,33.81 | IC5.40 139.41,37.81 v138.43,36.83 | 135.37,35.04 v135.89,35.56 | U1.10 155.6,36.42 v156.21,35.81 | v159.51,31.43 159.51,30.86 157.06,28.41 U1.27 | R40.1 129.29,14.73 127.13,14.73 127,14.86 | v130.68,14.86 130.3,15.24
  Top 0.254: R26.1 v113.85,6.92 114.05,6.73 | C21.1 151.13,26.67
  Top 0.305: U1.99 157.06,43.4 157.48,43.81 157.48,44.83 R7.1 | C20.1 171.58,40.77 171.24,40.42 U1.74 | U1.27 157.06,26.38 C25.1 | C21.1 C33.1
  Top 0.406: 135.37,34.81 135.37,35.04 | v148.59,20.32 148.59,21.34 151.13,23.88 C21.1
  Top 0.61: X4.2 150.11,36.83 C27.1
  Bottom 0.203: 163.45,34.8 162.56,34.8 160.15,37.21 154.56,37.21 152.02,39.75 145.41,39.75 143.51,37.85 143.51,35.57 142.86,34.92 | 154.94,36.07 159.26,36.07 160.02,35.31 160.02,31.94 v159.51,31.43 | 154.94,36.07 154.05,36.07 150.88,32.89 143,32.89 142.12,32.01 139.06,32.01 138.68,32.38 134.75,32.38 133.86,31.5 127.89,31.5 114.3,17.91 v114.3,15.24 | v155.57,26.04 155.76,26.23 v155.76,31.43 155.76,32.19 154.94,33.02 154.94,36.07
  other vias: 105.28,19.05 99.69,7.62 105.28,10.16 99.69,5.71 132.46,7.62 134.62,13.97 135.89,13.97 137.16,13.97 137.16,12.7 137.16,11.43 135.89,11.43 134.62,11.43 134.62,12.7 135.89,12.7 141.22,9.27 139.06,18.03 173.99,6.35 163.96,12.06 167.64,12.06 163.83,16.51 169.55,22.23 167.64,22.23 153.29,15.24 135.89,36.83 137.16,36.83 138.43,35.56 137.16,35.56 127.25,37.47 127.63,40.01 129.67,38.73 123.57,42.42 123.57,43.81 132.72,40.01 129.54,40.01 142.24,26.67 111.76,10.16 114.94,10.16 117.47,10.16 139.06,9.4 137.16,9.27 153.67,45.72 171.58,42.55 153.29,49.15 127.25,36.2 129.92,34.92 107.31,15.24 105.41,24.77 107.31,24.77 112.39,26.04 113.66,26.04 138.43,43.18 143.51,43.18 141.35,43.18 139.95,43.18 130.68,27.56 132.21,27.56 133.73,27.56 130.81,39.12 127.76,33.66 139.06,26.67 125.73,25.27 125.73,17.78 136.53,24.13 148.97,30.23 132.72,17.65 126.36,10.16 113.03,16.51 180.97,26.67 180.97,24.13 129.54,45.72 128.91,43.18 135.25,43.18 125.73,6.99 153.67,19.68 153.67,18.41 124.46,19.05 119.38,19.05 118.11,15.24 113.03,20.32 123.82,10.16 129.29,17.65 99.06,18.41 103.12,17.4 100.97,24.13 99.06,24.13 105.41,27.94 112.39,24.13 127.25,26.16 123.19,31.11 123.19,29.84 130.81,31.24 132.08,31.24 126.36,45.72 132.72,45.72 135.89,45.72 138.43,45.72 141.35,45.72 144.14,45.72 147.45,45.72 121.28,46.35 123.82,46.35 142.24,24.13 140.33,25.4 146.05,18.41 143,20.32 139.7,20.95 129.54,20.95 134.62,40.39 135.89,34.42 137.16,34.42 138.43,34.42 162.56,21.59 163.83,20.32 169.55,20.32 167.64,16.51 169.55,16.51 169.55,12.06 150.62,36.83 148.97,30.99 144.4,33.53 151.13,41.91 147.7,41.91 117.47,24.13 114.94,24.13 134.62,21.59 136.53,21.59 135.89,19.68 132.08,20.95 146.05,15.24 148.21,15.24 137.16,25.4 140.33,27.94 102.87,3.17 106.68,2.54 104.14,8.64 102.87,5.71 100.97,16.51 99.06,16.51 99.06,12.7 99.06,14.61 100.97,14.61 101.6,11.05 104.14,15.24 101.22,20.95 103.5,20.95 102.87,24.77 101.6,9.27 104.14,11.81 102.87,7.62 162.56,24.13 132.08,43.18
  pour Bottom (isolate 0.254, rank 6): 93.34,53.34 182.88,53.34 182.88,0 93.34,0
  pour Top (isolate 0.254, rank 6): 93.34,53.34 182.88,53.34 182.88,0 93.34,0
GREEN  (via drill 0.3 pad 0.64)
  Top 0.254: IC2.12 119.51,12.95 v119.38,13.08
  Top 0.305: v109.47,5.21 D22.-
  Bottom 0.305: v119.38,13.08 119.38,10.16 114.43,5.21 v109.47,5.21
GREEN1  (via drill 0.3 pad 0.64)
  Top 0.203: IC2.7 134.64,15.6 134.37,15.88 132.97,15.88 131.89,16.95 v120.02,16.95
  Top 0.305: v108.84,4.57 107.06,4.57 D21.-
  Bottom 0.305: v120.02,16.95 120.02,9.53 115.06,4.57 v108.84,4.57
I2C1_SCL  (via drill 0.3 pad 0.64)
  Top 0.203: v158.94,43.81 159.06,43.7 U1.95 159.06,41.98 162.24,38.8 162.24,36.89 161.75,36.4 161.75,32.7 163.33,31.11 166.37,31.11 172.47,25.02 172.47,12.95 173.99,11.43 175.89,11.43 176.53,12.06 176.53,13.97 J2.15 | J13.8 167.64,47.37 169.16,45.85 v169.16,44.45
  Bottom 0.203: v158.94,43.81 167.64,43.81 168.27,44.45 v169.16,44.45 | J13.8 167.64,51.44 166.24,52.83 102.11,52.83 J1.1
I2C1_SDA  (via drill 0.3 pad 0.64)
  Top 0.203: v158.12,43.81 158.56,43.37 U1.96 158.56,41.97 161.86,38.67 161.86,37.02 161.35,36.51 161.35,32.49 163.11,30.73 166.24,30.73 172.08,24.89 172.08,11.45 174.64,8.89 178.44,8.89 179.07,9.53 179.07,13.97 J2.22 | v168.66,43.81 168.53,43.94 168.53,45.97 165.1,49.4 J13.7 165.1,51.18 163.45,52.83 104.65,52.83 J1.2
  Bottom 0.203: v158.12,43.81 158.75,43.18 168.02,43.18 v168.66,43.81
ID
  Top 0.305: R19.2 102.74,16.64 99.08,20.3 J10.4
LED_LINK  (via drill 0.3 pad 0.64)
  Top 0.203: v123.32,26.04 114.94,26.04 114.68,26.29 114.68,27.94 R3.2 112.14,30.48 106.16,30.48 J7.10 | IC5.22 135.41,32.29 135.13,32 134.11,32 v132.97,30.86
  Bottom 0.203: v123.32,26.04 127.51,30.23 132.33,30.23 v132.97,30.86
LED_SPEED  (via drill 0.3 pad 0.64)
  Top 0.203: IC5.21 133.26,32.66 v133.1,32.83
  Bottom 0.203: v133.1,32.83 132.14,33.78 132.14,38.67 127.63,43.18 106.16,43.18 J7.11
N$1
  Top 0.305: J10.1 98.39,22.25 98.42,22.23 98.42,22.48
  Top 0.813: 107.44,21.97 C12.1 105.16,21.97 104.65,22.48 98.42,22.48 | 107.44,21.97 109.16,21.97 F1.1 | C11.1 107.44,21.97
N$2
  Top 0.203: R17.1 150.37,33.27 148.21,33.27 147.32,32.38 J12.6
N$3  (via drill 0.3 pad 0.64)
  Top 0.203: R5.1 v139.06,15.24 137.83,15.24 IC2.1 | v147.32,12.7 146.81,12.7 138.68,4.57 132.21,4.57 131.44,3.81 105.41,3.81 SW1.2 | IC2.3 136.64,15.99 v136.78,16.13
  Bottom 0.203: v147.32,12.7 141.6,12.7 v139.06,15.24 138.17,16.13 v136.78,16.13
N$4  (via drill 0.3 pad 0.64)
  Top 0.203: IC5.23 135.91,32.15 v135.19,31.43 | v155.96,8.26 v167.64,8.26
  Bottom 0.203: v135.19,31.43 135.19,27.88 135.64,27.43 136.94,27.43 142.15,22.23 154.14,22.23 154.94,21.42 154.94,13.34 155.96,12.32 v155.96,8.26 | v167.64,8.26 P1.2
N$5
  Top 0.254: IC2.9 131.6,14.45 131.57,14.48
  Top 0.305: R40.2 131.57,14.48 R12.1
N$6
  Top 0.203: J7.9 111.13,29.97 R2.2
N$7
  Top 0.203: J7.12 111.13,43.69 R4.2
N$8
  Top 0.203: D5.+ R1.1
N$9  (via drill 0.3 pad 0.64)
  Top 0.203: v136.65,26.8 X1.1
  Bottom 0.203: v136.65,26.8 137.03,26.8 141.99,21.84 153.99,21.84 154.56,21.28 154.56,13.08 155.57,12.06 155.57,9.27 154.94,8.64 154.94,6.99 153.42,5.46 P5.2
N$10
  Top 0.203: J8.1 98.2,10.57 98.42,10.79
  Top 0.305: 98.45,10.82 98.42,10.79
  Top 0.813: 107.44,13.08 C7.1 101.98,13.08 99.69,10.79 98.42,10.79 | F3.1 109.09,13.08 107.44,13.08 | 107.44,13.08 C8.1
N$12
  Top 0.305: IC2.14 112.28,11.95 R13.1
N$13
  Top 0.305: IC2.13 111.13,12.45 109.73,11.05 R14.1
N$15
  Top 0.203: D13.1 103.12,18.16 102.49,18.8 101.6,18.8 99.44,20.95 J10.3
  Top 0.305: R15.2 D13.1
N$18
  Top 0.305: PWR.- R26.2
N$22
  Top 0.203: D13.2 103.12,19.94 102.49,19.3 101.73,19.3 99.43,21.61 J10.2
  Top 0.305: R16.2 D13.2
N$23  (via drill 0.3 pad 0.64)
  Top 0.406: PWR.+ v122.55,7.49 | U2.2 125.22,23.88 125.09,23.75 | C18.2 137.67,22.73
  Top 0.61: C13.+ 135.89,22.73 136.02,22.61 135.38,22.61 C13.+ | C13.+ C18.2 137.79,22.73 R33.1 R35.2 | C13.+ 132.33,22.73 132.08,22.99 U2.TER U2.2 v124.33,23.88
  Bottom 0.406: v122.55,7.49 122.55,15.24 123.19,15.88 123.19,22.73 v124.33,23.88
  other vias: 128.91,24.77 132.72,24.77 132.72,22.86 130.81,22.86 130.81,24.77 128.91,22.86
  pour Top (isolate 0.254, no thermals): 132.72,21.59 128.91,21.59 arc-90 128.27,22.23 128.27,25.4 arc-90 128.91,26.04 132.72,26.04 arc-90 133.35,25.4 133.35,22.23 arc-90
  pour Bottom (isolate 0.254, no thermals): 132.72,21.59 128.91,21.59 arc-90 128.27,22.23 128.27,25.4 arc-90 128.91,26.04 132.72,26.04 arc-90 133.35,25.4 133.35,22.23 arc-90
N$24  (via drill 0.3 pad 0.64)
  Top 0.254: IC2.2 137.14,15.6 137.41,15.88 139.95,15.88 C31.2 R39.1
  Top 0.305: v140.21,19.68 R39.1
  Bottom 0.305: RST.T v140.21,19.68
N$25
  Top 0.305: IC2.15 132.23,11.45 R37.1
  Top 0.406: Q7.1 131.7,10.67 R37.1
N$26
  Top 0.305: R42.1 D22.+
N$27
  Top 0.406: R36.1 130.56,6.86 Q7.3
N$28
  Top 0.305: D21.+ R41.1
N$32
  Top 0.305: D23.- 112.65,5.08 118.24,5.08 119.08,5.92 135.85,5.92 136.14,6.22 IC2.21
N$33
  Top 0.305: R43.1 D23.+
N$34
  Top 0.305: IC2.4 136.14,16.7 C15.2 136.59,18.29 X2.2
N$37
  Top 0.305: IC2.5 135.64,16.57 C17.2 135.06,18.29 X2.1
N$56  (via drill 0.3 pad 0.64)
  Top 0.203: U3.2 v111.76,40.01 | v116.97,29.46 R61.2
  Bottom 0.203: v116.97,29.46 116.33,30.1 114.3,30.1 112.39,32 112.39,39.37 v111.76,40.01
N$58  (via drill 0.3 pad 0.64)
  Top 0.203: R60.2 v115.44,29.46 | U3.7 v111.76,33.66
  Bottom 0.203: v115.44,29.46 114.05,29.46 113.09,30.42 113.03,30.48 111.76,31.75 v111.76,33.66
N$59
  Top 0.305: R60.1 R61.1 118.43,27.18 C10.2
N$123
  Top 0.203: R59.1 132.72,33.78 133.1,33.4 133.73,33.4 133.82,33.31 IC5.20
N$127
  Top 0.203: IC5.32 140.62,33.81 141.1,34.29 141.1,35.05 141.35,35.31 R58.2
OTG_FS_DM  (via drill 0.3 pad 0.64)
  Top 0.203: U1.70 169.11,38.42 166.75,36.07 165.74,36.07 v164.08,34.42 | v110.49,19.56 109.98,19.56 R16.1
  Bottom 0.203: v110.49,19.56 110.87,19.18 114.55,19.18 127.63,32.26 133.48,32.26 134.37,33.15 139.19,33.15 139.6,32.74 141.71,32.74 143.89,34.92 143.89,37.72 145.54,39.37 151.89,39.37 154.43,36.83 159.89,36.83 162.56,34.16 163.83,34.16 v164.08,34.42
OTG_FS_DP  (via drill 0.3 pad 0.64)
  Top 0.203: U1.71 169.1,38.92 166.75,36.58 165.35,36.58 163.44,34.67 163.44,34.04 163.96,33.53 v164.08,33.53 | v110.49,18.54 109.98,18.54 R15.1
  Bottom 0.203: v110.49,18.54 110.74,18.8 114.68,18.8 127.76,31.88 133.6,31.88 134.49,32.77 138.94,32.77 139.33,32.37 141.85,32.37 144.27,34.8 144.27,37.59 145.67,38.99 151.76,38.99 154.31,36.45 159.77,36.45 162.43,33.78 163.83,33.78 v164.08,33.53
PA0/WKUP
  Top 0.203: U1.23 155.62,29.93 155.83,29.72 155.83,28.7 152.4,25.27 152.4,24.32 149.35,21.27 149.35,18.29 148.84,17.78 148.84,12.7 147.95,11.81 146.43,11.81 138.81,4.19 133.73,4.19 J5.1
PA3
  Top 0.203: J5.2 135.89,3.81 138.94,3.81 146.3,11.18 149.4,11.18 150.5,12.27 150.5,20.7 154.05,24.26 154.05,25.4 155.83,27.18 U1.26
PA4
  Top 0.203: U1.29 158.06,24.33 155.96,22.23 152.6,22.23 150.88,20.5 150.88,12.08 149.34,10.54 146.18,10.54 139.06,3.43 138.05,3.43 J5.3
PA5
  Top 0.203: U1.30 158.56,24.32 156.08,21.84 152.74,21.84 151.26,20.36 151.26,8 147.83,4.57 141.73,4.57 J5.4
PA6
  Top 0.203: U1.31 159.06,24.31 156.21,21.46 152.89,21.46 151.64,20.21 151.64,7.87 147.95,4.19 143.89,4.19 J5.5
PA8  (via drill 0.3 pad 0.64)
  Top 0.203: U1.67 172.37,36.92 172.72,36.58 v172.72,35.56
  Bottom 0.203: v172.72,35.56 172.08,34.92 171.2,34.92 169.8,36.32 165.61,36.32 162.05,39.88 156.34,39.88 147.32,48.9 133.99,48.9 J4.6
PA9  (via drill 0.3 pad 0.64)
  Top 0.203: U1.68 169.12,37.42 168.34,36.64 v168.34,35.56 | v164.59,5.08 157.48,5.08 J6.1 153.67,1.27 130.81,1.27 130.18,1.91 v130.18,2.54 | v127.76,15.49 R18.1
  Bottom 0.203: v168.34,35.56 168.34,34.48 168.5,34.32 168.5,33.23 168.49,33.23 167.89,32.64 165.35,32.64 164.34,31.62 162.31,31.62 160.53,29.84 160.53,9.14 v164.59,5.08 | v130.18,2.54 130.18,13.08 v127.76,15.49
PA10  (via drill 0.3 pad 0.64)
  Top 0.203: U1.69 169.12,37.92 167.77,36.58 v167.77,34.92 | v164.08,4.45 159.38,4.45 J6.2 155.83,0.89 v107.95,0.89 | v107.95,16.64 R19.1
  Bottom 0.203: v167.77,34.92 167.77,34.42 168.05,34.14 168.05,33.36 167.7,33.02 165.1,33.02 164.08,32 162.05,32 160.15,30.1 160.15,8.38 v164.08,4.45 | v107.95,0.89 v107.95,16.64
PB0
  Top 0.203: U1.35 161.06,25.8 156.34,21.08 153.03,21.08 152.02,20.07 152.02,7.75 148.08,3.81 146.05,3.81 J5.6
PB1
  Top 0.203: U1.36 161.56,25.8 156.46,20.7 153.19,20.7 152.4,19.91 152.4,7.62 J5.7
PB14  (via drill 0.3 pad 0.64)
  Top 0.203: U1.53 169.59,29.93 166.18,33.34 v166.18,33.66
  Bottom 0.203: v166.18,33.66 165.99,33.85 165.99,34.6 165.48,35.12 165.29,35.12 161.67,38.73 155.57,38.73 147.32,46.99 124.21,46.99 J1.9
PB15  (via drill 0.3 pad 0.64)
  Top 0.203: U1.54 169.6,30.43 166.75,33.27 166.75,34.29 v166.62,34.42
  Bottom 0.203: v166.62,34.42 166.62,34.54 165.67,35.5 165.42,35.5 161.8,39.12 155.83,39.12 147.32,47.62 126.11,47.62 J1.10
PC0  (via drill 0.3 pad 0.64)
  Top 0.203: U1.15 155.94,33.92 v156.21,33.66
  Bottom 0.203: v156.21,33.66 156.21,33.02 156.97,32.26 156.97,14.1 156.59,13.72 156.59,6.73 154.56,4.7 P5.1 J5.8
PC13  (via drill 0.3 pad 0.64)
  Top 0.203: U1.7 156,37.92 156.84,37.08 156.84,35.18 v156.21,34.54 | v156.97,5.71 165.1,5.71 167.64,3.17 J6.6
  Bottom 0.203: P1.1 J6.6 | v156.21,34.54 156.84,33.91 156.84,33.02 157.35,32.51 157.35,13.97 156.97,13.59 v156.97,5.71
PD3  (via drill 0.3 pad 0.64)
  Top 0.203: 164.81,41.37 v164.91,41.27 164.59,41.59 164.59,42.74 164.56,42.7 U1.84 164.56,44.74 160.53,48.77 154.92,48.77 153.67,50.01 153.67,51.44 153.03,52.07 130.81,52.07 J4.7
  Bottom 0.203: J2.4 173.35,41.27 v164.91,41.27
PD6  (via drill 0.3 pad 0.64)
  Top 0.203: U1.87 v163.06,44.45 163.06,45.6 160.27,48.39 129.41,48.39 J4.8
  Bottom 0.203: v163.06,44.45 167,44.45 168.27,45.72 J2.3
PD11
  Top 0.203: J2.35 179.45,46.61 179.45,32.77 178.44,31.75 173.99,31.75 173.31,32.42 U1.58
  Bottom 0.203: J4.3 140.97,52.07 163.19,52.07 163.83,51.44 163.83,49.53 166.37,46.99 176.53,46.99 J2.35
PD12
  Top 0.203: J2.2 176.53,46.99 178.44,46.99 179.07,46.35 179.07,34.92 178.44,34.29 174.75,34.29 173.39,32.92 U1.59
  Bottom 0.203: J2.2 167.64,48.26 166.37,49.53 166.37,51.82 165.74,52.45 138.81,52.45 J4.4
PD13  (via drill 0.3 pad 0.64)
  Top 0.203: v132.84,49.02 J4.5 | U1.60 167.68,33.42 v167.45,33.66
  Bottom 0.203: 167.39,33.72 v167.45,33.66 167.19,33.91 167.19,34.73 166.05,35.88 165.55,35.88 161.93,39.5 156.08,39.5 147.32,48.26 133.6,48.26 v132.84,49.02
PE2  (via drill 0.3 pad 0.64)
  Top 0.203: U1.1 155.54,40.92 159.45,37.02 159.45,34.48 v159.26,34.29 | 162.11,12.06 162.12,12.06 | 162.12,12.06 162.18,12.13 | v158.75,12.64 159.51,11.87 J9.2 161.92,11.87 162.12,12.06
  Bottom 0.203: v158.75,12.64 158.75,12.83 158.88,12.95 158.88,33.91 v159.26,34.29
PE3  (via drill 0.3 pad 0.64)
  Top 0.203: U1.2 155.54,40.42 158.88,37.08 v158.88,35.43
  Bottom 0.203: J12.3 146.05,24.13 155.57,24.13 156.59,25.15 156.59,32 155.57,33.02 155.57,34.8 155.96,35.18 158.62,35.18 v158.88,35.43
PE4  (via drill 0.3 pad 0.64)
  Top 0.203: U1.3 155.53,39.92 158.24,37.21 158.24,34.92 158.62,34.54 158.62,33.66 158.18,33.21 v157.48,33.21
  Bottom 0.203: J6.3 160.02,6.6 157.35,9.27 157.35,13.34 157.73,13.72 157.73,32.96 v157.48,33.21
PE5  (via drill 0.3 pad 0.64)
  Top 0.203: U1.4 155.52,39.42 157.73,37.21 157.73,34.16 v157.86,34.04
  Bottom 0.203: J6.4 162.56,4.57 157.73,9.4 157.73,13.08 158.12,13.46 158.12,33.78 v157.86,34.04
PE6  (via drill 0.3 pad 0.64)
  Top 0.203: U1.5 155.51,38.92 157.23,37.21 157.23,34.67 v157.1,34.54
  Bottom 0.203: J6.5 158.12,9.52 158.12,12.96 158.5,13.34 158.5,34.29 158.12,34.67 157.23,34.67 v157.1,34.54
PFBOUT  (via drill 0.3 pad 0.64)
  Top 0.152: IC5.19 134.24,33.78
  Top 0.203: 133.03,34.61 132.97,34.67 | IC5.16 133.61,35.31 132.97,34.67 | 134.24,33.78 133.35,33.78 132.97,34.16 132.97,34.67 | IC5.30 141.88,32.66 C50.1 v141.32,33.44 v141.31,33.44 141.91,34.04 C54.2
  Top 0.406: 132.97,34.67 v132.72,34.67 131.57,34.67 C53.2 129.22,33.78 C55.+
  Bottom 0.406: v132.72,34.67 132.72,34.16 133.22,33.66 141.1,33.66 v141.31,33.44
RD+
  Top 0.203: U3.14 R10.2 125.35,39.75 126.24,39.75 128.68,37.31 IC5.12
RD-
  Top 0.203: U3.16 R11.1 125.35,40.26 126.36,40.26 128.81,37.81 IC5.11
RESET  (via drill 0.3 pad 0.64)
  Top 0.203: U1.14 v153.31,34.42 152.79,34.42 R24.1 | IC2.8 133.29,15.05 132.02,16.32 v122.3,16.32 v120.65,16.32
  Bottom 0.203: v122.3,16.32 122.3,23.01 129.14,29.84 132.96,29.84 134.49,31.38 134.49,31.62 134.87,32 137.16,32 137.54,31.62 142.37,31.62 143.26,32.51 151.39,32.51 v153.31,34.42
  Bottom 0.305: v120.65,16.32 120.65,8.89 J11.3
RX+
  Top 0.203: U3.3 109.96,38.73 arc45 109.78,38.66 109.29,38.17 arc45 109.22,37.99 109.22,37.08 arc90 109.47,36.83 109.6,36.83 arc-90 109.85,36.58 109.85,36.45 arc-90 109.6,36.2 109.38,36.2 arc45 108.48,35.82 108.05,35.39 arc-45 107.82,35.3 J7.3
RX-
  Top 0.203: U3.1 109.32,41.27 arc45 109.15,41.2 108.66,40.71 arc45 108.58,40.53 108.58,38.84 arc-45 108.51,38.66 108.28,38.43 arc-45 108.1,38.36 J7.6
SDIO_CK  (via drill 0.3 pad 0.64)
  Top 0.203: U1.80 166.56,45.53 v164.21,47.88
  Bottom 0.203: v164.21,47.88 161.54,47.88 160.02,49.4 J13.5
SDIO_CMD  (via drill 0.3 pad 0.64)
  Top 0.203: U1.83 165.06,46.01 v162.56,48.51
  Bottom 0.203: v162.56,48.51 J13.6
SDIO_D0  (via drill 0.3 pad 0.64)
  Top 0.203: 170.36,35.88 U1.65 170.37,35.87 171.14,35.87 v171.45,35.56
  Bottom 0.203: v171.45,35.56 170.31,36.7 165.74,36.7 162.18,40.26 156.59,40.26 151.76,45.09 151.76,48.9 J13.1
SDIO_D1  (via drill 0.3 pad 0.64)
  Top 0.203: U1.66 171.85,36.42 v172.08,36.2
  Bottom 0.203: v172.08,36.2 171.2,37.08 165.86,37.08 162.31,40.64 156.84,40.64 152.4,45.09 J13.2
SDIO_D2
  Top 0.203: J13.3 156.21,52.07 160.66,52.07 161.29,51.44 161.29,50.16 161.93,49.53 163.96,49.53 167.56,45.93 U1.78
SDIO_D3
  Top 0.203: U1.79 167.06,45.9 163.81,49.15 159.13,49.15 J13.4
SPI2_MISO  (via drill 0.3 pad 0.64)
  Top 0.203: 153.76,32.86 v153.67,32.77 153.83,32.92 U1.17 156.05,32.92 156.84,32.13 156.84,28.7 153.67,25.53 153.67,24.45 150.11,20.89 150.11,17.4 v149.86,17.14 | v153.67,17.14 161.93,17.14 | 161.93,17.14 162.08,17.14 | J9.7 161.7,17.37 161.93,17.14
  Bottom 0.203: v149.86,17.14 v153.67,17.14 | J12.1 146.05,31.75 152.65,31.75 v153.67,32.77
SPI2_MOSI  (via drill 0.3 pad 0.64)
  Top 0.203: U1.18 155.92,32.42 156.46,31.88 156.46,28.83 153.03,25.4 v153.03,24.77 153.03,24.38 149.73,21.08 149.73,18.03 149.22,17.53 149.22,13.34 v149.86,12.7 | v153.67,12.7 154.18,13.21 162.07,13.21 161.83,12.97 J9.3 161.67,12.95 161.93,12.7 162.03,12.7
  Bottom 0.203: v149.86,12.7 v153.67,12.7 | v153.03,24.77 149.22,24.77 148.59,25.4 148.59,26.67 J12.5
SPI2_SCK  (via drill 0.3 pad 0.64)
  Top 0.203: U1.47 167.06,27.3 167.07,27.3 | U1.47 | U1.47 167.13,27.1 167.13,24.26 165.1,22.23 165.1,16.51 163.76,15.17 J9.5 162.11,15.17 162.18,15.24 | v156.4,15.24 162.18,15.24 | 162.18,15.24 162.24,15.24
  Bottom 0.203: v156.4,15.24 156.4,22.96 155.8,23.56 152.59,23.56 144.72,23.56 143.51,24.77 143.51,26.67 J12.2
SPI3_MISO  (via drill 0.3 pad 0.64)
  Top 0.203: U1.90 161.56,45.91 159.84,47.62 117.22,47.62 v116.59,46.99
  Bottom 0.203: v116.59,46.99 J1.6
SPI3_MOSI  (via drill 0.3 pad 0.64)
  Top 0.203: U1.91 161.06,45.85 159.67,47.24 119.38,47.24 v119.13,46.99
  Bottom 0.203: v119.13,46.99 J1.7
SPI3_NSS
  Top 0.203: U1.77 168.06,45.94 163.83,50.16 163.83,51.82 163.19,52.45 119.51,52.45 J1.8
SPI3_SCK
  Top 0.203: U1.89 162.06,46.01 160.06,48.01 115.7,48.01 | 115.7,48.01 115.44,48.01 | 115.44,48.01 113.03,48.01 J1.5 | D5.- 115.57,47.88 | 115.57,47.88 115.7,48.01 | 115.57,47.88 115.44,48.01
SWCLK  (via drill 0.3 pad 0.64)
  Top 0.203: U1.76 168.56,39.4 166.56,37.4 165.15,37.4 162.56,34.81 162.56,33.4 v162.81,33.15 | R45.2 133.35,8.51 v133.35,10.16 133.35,10.76 IC2.16 | v158.75,10.79 v153.03,10.79
  Bottom 0.203: v162.81,33.15 162.06,33.15 159.32,30.41 159.32,11.37 v158.75,10.79 | v153.03,10.79 133.99,10.79 v133.35,10.16
SWDIO  (via drill 0.3 pad 0.64)
  Top 0.203: U1.72 169.09,39.42 166.62,36.96 165.21,36.96 163.02,34.76 163.02,33.83 163.45,33.4 v163.45,32.64 | v159.38,10.16 v153.67,10.16
  Top 0.305: IC2.17 v134.14,9.53 134.14,8.99 R44.1
  Bottom 0.203: v159.38,10.16 159.7,10.48 159.7,30.21 162,32.51 163.32,32.51 v163.45,32.64 | v153.67,10.16 134.78,10.16 v134.14,9.53
TD+
  Top 0.203: U3.9 R8.2 125.35,33.4 126.49,33.4 128.9,35.81 IC5.15
TD-
  Top 0.203: U3.11 R9.1 125.35,33.91 126.36,33.91 128.77,36.31 IC5.14
TGT_3V3  (via drill 0.3 pad 0.64)
  Top 0.203: IC2.6 135.14,15.99 v135,16.13 134.87,16.26 133.1,16.26 C30.2
  Top 0.254: R43.2 109.47,6.73 107.31,6.73 | 107.31,6.73 104.9,6.73 R41.2 | R42.2 107.19,6.6 107.31,6.73
  Top 0.305: IC2.29 139.83,12.95 C29.2
  Top 0.406: R43.2 111.82,4.38 v130.81,4.38 | v138.94,6.86 140.33,8.26 C1.2 140.33,12.45 C29.2 R5.2 v142.88,14.1 | v135.51,6.86 R44.2 | R37.2 130.05,9.4 130.05,9.27 | 130.05,9.27 Q7.2 129.67,8.89 | 139.19,22.73 R33.2 141.73,20.32 R39.2 v142.88,17.14 | 130.05,9.27 130.05,9.02 v130.81,8.26
  Bottom 0.406: v130.81,4.38 130.81,6.48 | 130.81,6.48 130.81,6.86 | 130.81,6.86 130.81,7.24 | 130.81,7.24 v130.81,8.26 | v138.94,6.86 v135.51,6.86 131.19,6.86 | 131.19,6.86 130.81,6.86 | 130.81,7.24 131.19,6.86 | 131.19,6.86 130.81,6.48 | v142.88,14.1 v142.88,17.14 | v142.88,17.14 136.02,17.14 v135,16.13 | I_3V3.T v142.88,17.14
TGT_D+
  Top 0.203: D11.1 102.87,9.27 102.23,9.91 100.97,9.91 100.39,9.34 100.33,9.27 J8.3
  Top 0.305: D11.1 R13.2 108.97,8.38 R36.2
TGT_D-
  Top 0.203: D11.2 102.87,11.05 102.23,10.41 100.71,10.41 100.22,9.92 J8.2
  Top 0.305: R14.2 D11.2
TX+
  Top 0.203: U3.8 110.11,32.38 arc90 109.85,32.13 109.85,31.37 arc-90 109.6,31.11 109.47,31.11 arc-90 109.22,31.37 109.22,33.17 arc45 109.15,33.35 108.91,33.58 arc45 108.73,33.66 106.95,33.66 J7.1
TX-
  Top 0.203: J7.2 108.16,34.28 arc45 108.87,34.57 109.15,34.85 arc-45 109.32,34.92 109.6,34.92 arc-90 109.85,34.67 109.85,33.91 arc90 110.11,33.66 110.24,33.66 arc90 110.49,33.91 110.49,34.67 arc-90 110.74,34.92 U3.6
USART1_RX  (via drill 0.3 pad 0.64)
  Top 0.203: U1.93 160.06,45.64 159.22,46.48 151.64,46.48 v151.13,45.97
  Bottom 0.203: J4.1 147.32,50.8 151.13,46.99 v151.13,45.97
USART1_TX  (via drill 0.3 pad 0.64)
  Top 0.203: U1.92 160.56,45.74 159.44,46.86 150.75,46.86 v150.5,46.61
  Bottom 0.203: v150.5,46.61 147.57,49.53 143.51,49.53 J4.2
USART6_RX  (via drill 0.3 pad 0.64)
  Top 0.203: U1.64 169.3,35.42 v169.16,35.56 | v165.1,6.99 167.64,4.45 170.81,4.45 J6.8
  Bottom 0.203: v169.16,35.56 169.55,35.18 169.55,33.02 168.4,31.88 165.86,31.88 164.85,30.86 162.81,30.86 161.29,29.34 161.29,10.79 v165.1,6.99 | J6.8 172.72,4.32 P10.1 172.72,5.33
USART6_TX  (via drill 0.3 pad 0.64)
  Top 0.203: U1.63 169.04,34.92 v168.91,34.8 | v164.46,6.35 165.1,6.35 167.64,3.81 168.91,3.81 J6.7
  Bottom 0.203: v168.91,34.8 168.92,34.79 168.92,33.03 168.91,33.03 168.91,33.02 168.15,32.26 165.61,32.26 164.59,31.24 162.56,31.24 160.91,29.59 160.91,9.91 v164.46,6.35 | J6.7 170.18,4.32 P9.2 170.18,5.33
USB5V  (via drill 0.3 pad 0.64, 0.38 pad 0.81)
  Top 0.813: U2.3 C14.+ 112.2,21.59 | R12.2 R18.2 v127.63,13.97 113.54,13.97 111.76,15.75 | 112.2,21.59 v111.76,21.59 | 111.76,15.75 111.76,16.26 | 111.76,16.26 111.76,21.08 | 111.76,21.08 v111.76,21.59 | v111.76,21.59 111.76,22.04 | 111.76,22.04 F1.2 | F3.2 111.25,15.75 | 111.25,15.75 111.76,15.75 | 111.25,15.75 111.76,16.26 | 111.76,22.04 112.2,21.59 | 112.2,21.59 112.2,21.53 111.76,21.08
  Bottom 0.406: 5V.T v111.76,21.59
  Bottom 0.813: J2.1 J2.36 179.45,49.15 179.45,6.73 178.44,5.71 175.89,5.71 174.62,4.45 174.62,1.91 173.74,1.02 129.79,1.02 | 129.79,1.02 129.03,1.02 | 129.03,1.02 128.27,1.02 | 128.27,1.02 120.9,1.02 J11.5 | v127.63,13.97 129.03,12.57 129.03,1.78 | 129.03,1.78 129.03,1.02 | 128.27,1.02 129.03,1.78 | 129.03,1.78 129.79,1.02
VCAP1
  Top 0.203: U1.49 168.06,25.06 C23.2
VCAP2
  Top 0.305: U1.73 172,39.92 172.72,40.64 172.72,45.59 C24.2
VDDA
  Top 0.203: R25.2 153.42,30.35 154.74,30.35 U1.22
  Top 0.305: R25.2 C33.2 C21.2 L2.1
XTALIN
  Top 0.203: U1.12 153.81,35.42 153.03,36.2 153.03,37.85 152.85,38.03 X4.1 149.93,38.03 C27.2
XTALOUT
  Top 0.203: U1.13 153.67,34.92 152.97,35.63 X4.3 150.31,35.63 149.86,35.18 C28.2

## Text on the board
tPlace: LOCK | OPEN
bPlace: 5V | 5V | PB_8 | PB_9 | AREF | GND | PB_3 | PB_4 | PB_5 | PA_8 | PB_6 | PB_7 | PC_9 | PD_2 | PB_9 | PB_8 | D12 | D11 | PA_15 | PB_14 | PB_15 | PD_6 | PD_3 | PD_13 | PD_12 | PD_11 | PC_8 | PC_10 | PC_11 | PC_12 | D6 | E0 | D3 | E1 | D7 | GND | D4 | D5 | D0 | D15 | SPI | D2 | D1 | PC_2 | 3V3/NC | E7 | D5 | PB_10 | PC_3 | E9 | E10 | PE_3 | GND | E11 | E12 | E13 | E14 | D8 | E15 | V1.1 | PB_10 | SD_SCK | D9 | D10 | PC_2 | SD_MISO | B8 | B9 | Innovate with China | PC_3 | SD_MOSI | BT0 | BT1 | www.seeedstudio.com | PE_2 | SD_CS | 3V3 | 3V3 | ANALOG IN | GND | GND | NC | 3V3 | RST | 3V3 | 5V | GND | GND | NC | PA_0 | PA_3 | PA_4 | PA_5 | PA_6 | PB_0 | PB_1 | PC_0 | PA_9 | PA_10 | PE_3 | PE_5 | PE_6 | PC_13 | PC_6 | PC_7
tValues: Micro USB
